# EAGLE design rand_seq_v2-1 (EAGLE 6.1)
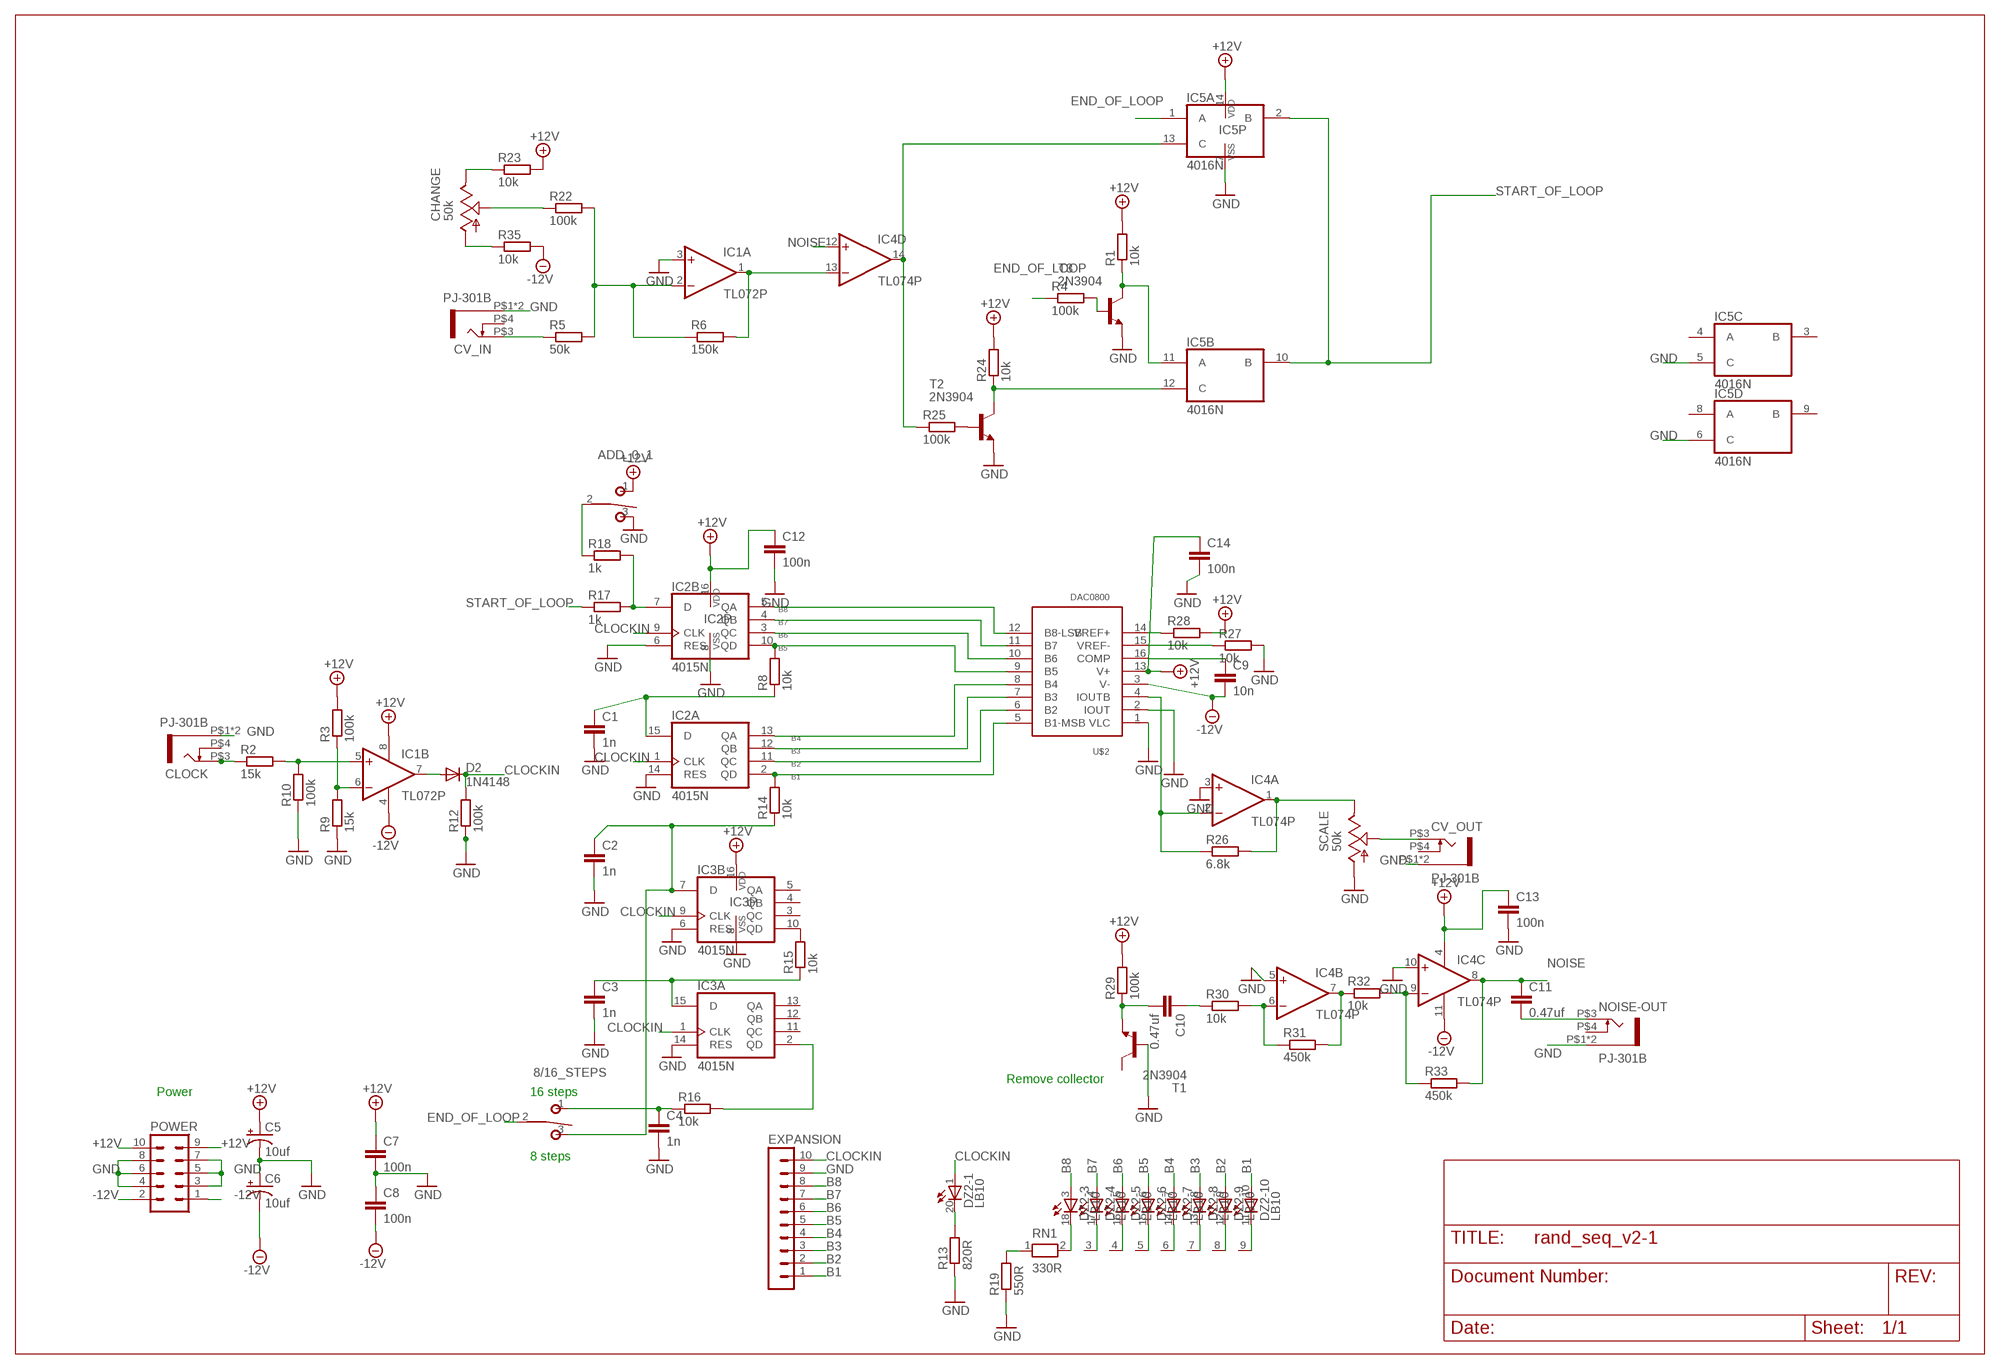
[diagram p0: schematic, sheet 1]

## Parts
8/16_STEPS  T-80-T-SPDT  [M9040P]
ADD_0_1  T-80-T-SPDT-ON-OFF-ON  [M9040P]
C1  1n  C-EU025-024X044  [C025-024X044]
C2  1n  C-EU025-024X044  [C025-024X044]
C3  1n  C-EU025-024X044  [C025-024X044]
C4  1n  C-EU025-024X044  [C025-024X044]
C5  10uf  CAP_POLPTH2  [CPOL-RADIAL-10UF-25V]
C6  10uf  CAP_POLPTH2  [CPOL-RADIAL-10UF-25V]
C7  100n  C-EU050-024X044  [C050-024X044]
C8  100n  C-EU050-024X044  [C050-024X044]
C9  10n  C-EU025-024X044  [C025-024X044]
C10  0.47uf  C-EU050-035X075  [C050-035X075]
C11  0.47uf  C-EU050-035X075  [C050-035X075]
C12  100n  C-EU050-024X044  [C050-024X044]
C13  100n  C-EU050-024X044  [C050-024X044]
C14  100n  C-EU050-024X044  [C050-024X044]
CHANGE  50k  ALPHA-9MMF2A  [EVUF]
CLOCK  PJ-301B  [PJ-301B]
CV_IN  PJ-301B  [PJ-301B]
CV_OUT  PJ-301B  [PJ-301B]
D2  1N4148  1N4148DO35-7  [DO35-7]
DZ2  LB10  [LB10]
EXPANSION  MA10-1  [MA10-1]
IC1  TL072P  [DIL08]
IC2  4015N  [DIL16]
IC3  4015N  [DIL16]
IC4  TL074P  [DIL14]
IC5  4016N  [DIL14]
NOISE-OUT  PJ-301B  [PJ-301B]
POWER  10_PIN_HEADER  [MA05-2]
R1  10k  R-EU_0207/10  [0207/10]
R2  15k  R-EU_0207/10  [0207/10]
R3  100k  R-EU_0207/10  [0207/10]
R4  100k  R-EU_0207/10  [0207/10]
R5  50k  R-EU_0207/10  [0207/10]
R6  150k  R-EU_0207/10  [0207/10]
R8  10k  R-EU_0207/10  [0207/10]
R9  15k  R-EU_0207/10  [0207/10]
R10  100k  R-EU_0207/10  [0207/10]
R12  100k  R-EU_0207/10  [0207/10]
R13  820R  R-EU_0207/10  [0207/10]
R14  10k  R-EU_0207/10  [0207/10]
R15  10k  R-EU_0207/10  [0207/10]
R16  10k  R-EU_0207/10  [0207/10]
R17  1k  R-EU_0207/10  [0207/10]
R18  1k  R-EU_0207/10  [0207/10]
R19  550R  R-EU_0207/2V  [0207/2V]
R22  100k  R-EU_0207/10  [0207/10]
R23  10k  R-EU_0207/10  [0207/10]
R24  10k  R-EU_0207/10  [0207/10]
R25  100k  R-EU_0207/10  [0207/10]
R26  6.8k  R-EU_0207/10  [0207/10]
R27  10k  R-EU_0207/10  [0207/10]
R28  10k  R-EU_0207/10  [0207/10]
R29  100k  R-EU_0207/10  [0207/10]
R30  10k  R-EU_0207/10  [0207/10]
R31  450k  R-EU_0207/10  [0207/10]
R32  10k  R-EU_0207/10  [0207/10]
R33  450k  R-EU_0207/10  [0207/10]
R35  10k  R-EU_0207/10  [0207/10]
RN1  330R  RN08  [RN-9]
SCALE  50k  ALPHA-9MMF2A  [EVUF]
T1  2N3904  [TO92]
T2  2N3904  [TO92]
T3  2N3904  [TO92]
U$2  DAC0800  [DIL16]

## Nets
+12V [power]: ADD_0_1.1(O) C5.1(+) C7.1 C12.1 C13.1 C14.1 IC1.8(P:V+) IC2.16(P:VDD) IC3.16(P:VDD) IC4.4(P:V+) IC5.14(P:VDD) POWER.9 POWER.10 R1.2 R3.2 R23.2 R24.2 R28.2 R29.2 U$2.13(V+)
-12V [power]: C6.2(-) C8.2 C9.2 IC1.4(P:V-) IC4.11(P:V-) POWER.1 POWER.2 R35.2 U$2.3(V-)
B1: DZ2.10(-10:A) EXPANSION.1 IC2.2(A:QD) R14.2 U$2.5(B1-MSB)
B2: DZ2.9(-9:A) EXPANSION.2 IC2.11(A:QC) U$2.6(B2)
B3: DZ2.8(-8:A) EXPANSION.3 IC2.12(A:QB) U$2.7(B3)
B4: DZ2.7(-7:A) EXPANSION.4 IC2.13(A:QA) U$2.8(B4)
B5: DZ2.6(-6:A) EXPANSION.5 IC2.10(B:QD) R8.2 U$2.9(B5)
B6: DZ2.5(-5:A) EXPANSION.6 IC2.3(B:QC) U$2.10(B6)
B7: DZ2.4(-4:A) EXPANSION.7 IC2.4(B:QB) U$2.11(B7)
B8: DZ2.3(-3:A) EXPANSION.8 IC2.5(B:QA) U$2.12(B8-LSB)
CLOCKIN: D2.C DZ2.1(-1:A) EXPANSION.10 IC2.1(A:CLK) IC2.9(B:CLK) IC3.1(A:CLK) IC3.9(B:CLK) R12.2
END_OF_LOOP: 8/16_STEPS.2(P) IC5.1(A:A) R4.1
GND [ground]: ADD_0_1.3(S) C1.2 C2.2 C3.2 C4.2 C5.2(-) C6.1(+) C7.2 C8.1 C12.2 C13.2 C14.2 CLOCK.P$1 CLOCK.P$2 CV_IN.P$1 CV_IN.P$2 CV_OUT.P$1 CV_OUT.P$2 EXPANSION.9 IC1.3(A:+IN) IC2.6(B:RES) IC2.8(P:VSS) IC2.14(A:RES) IC3.6(B:RES) IC3.8(P:VSS) IC3.14(A:RES) IC4.3(A:+IN) IC4.5(B:+IN) IC4.10(C:+IN) IC5.5(C:C) IC5.6(D:C) IC5.7(P:VSS) NOISE-OUT.P$1 NOISE-OUT.P$2 POWER.3 POWER.4 POWER.5 POWER.6 POWER.7 POWER.8 R9.1 R10.1 R12.1 R13.1 R19.1 R27.2 SCALE.1(A) T1.2(B) T2.3(E) T3.3(E) U$2.1(VLC) U$2.2(IOUT)
MAIN_OUT: IC4.1(A:OUT) R26.2 SCALE.3(E)
N$1: R4.2 T3.2(B)
N$2: CLOCK.P$3 R2.1
N$3: CV_IN.P$3 R5.1
N$4: IC5.11(B:A) R1.1 T3.1(C)
N$5: IC1.5(B:+IN) R2.2 R10.2
N$6: IC1.2(A:-IN) R5.2 R6.1 R22.2
N$7: IC1.1(A:OUT) IC4.13(D:-IN) R6.2
N$8: D2.A IC1.7(B:OUT)
N$9: 8/16_STEPS.3(S) C2.1 IC3.7(B:D) R14.1
N$10: C1.1 IC2.15(A:D) R8.1
N$11: ADD_0_1.2(P) R18.1
N$12: IC1.6(B:-IN) R3.1 R9.2
N$13: IC4.2(A:-IN) R26.1 U$2.4(IOUTB)
N$14: IC3.10(B:QD) R15.2
N$15: C11.2 NOISE-OUT.P$3
N$16: C10.2 R29.1 T1.3(E)
N$17: 8/16_STEPS.1(O) C4.1 R16.1
N$18: C3.1 IC3.15(A:D) R15.1
N$19: IC2.7(B:D) R17.2 R18.2
N$20: C10.1 R30.1
N$21: IC4.6(B:-IN) R30.2 R31.1
N$22: IC4.7(B:OUT) R31.2 R32.1
N$23: R27.1 U$2.15(VREF-)
N$24: IC4.14(D:OUT) IC5.13(A:C) R25.1
N$25: C9.1 U$2.16(COMP)
N$26: R28.1 U$2.14(VREF+)
N$27: IC4.9(C:-IN) R32.2 R33.1
N$28: DZ2.20(-1:C) R13.2
N$29: IC3.2(A:QD) R16.2
N$30: DZ2.18(-3:C) RN1.2
N$31: DZ2.17(-4:C) RN1.3
N$32: DZ2.16(-5:C) RN1.4
N$33: DZ2.15(-6:C) RN1.5
N$34: DZ2.14(-7:C) RN1.6
N$35: DZ2.13(-8:C) RN1.7
N$36: DZ2.12(-9:C) RN1.8
N$37: DZ2.11(-10:C) RN1.9
N$38: R19.2 RN1.1
N$39: CV_OUT.P$3 SCALE.2(S)
N$43: CHANGE.2(S) R22.1
N$44: R25.2 T2.2(B)
N$45: IC5.12(B:C) R24.1 T2.1(C)
N$47: CHANGE.3(E) R23.1
N$48: CHANGE.1(A) R35.1
NOISE: C11.1 IC4.8(C:OUT) IC4.12(D:+IN) R33.2
START_OF_LOOP: IC5.2(A:B) IC5.10(B:B) R17.1
Unconnected: CLOCK.P$4 CV_IN.P$4 CV_OUT.P$4 DZ2.2(-2:A) DZ2.19(-2:C) IC3.3(B:QC) IC3.4(B:QB) IC3.5(B:QA) IC3.11(A:QC) IC3.12(A:QB) IC3.13(A:QA) IC5.3(C:B) IC5.4(C:A) IC5.8(D:A) IC5.9(D:B) NOISE-OUT.P$4 T1.1(C)

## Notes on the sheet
- /Users/aash/Dropbox/Electronics/!MODULAR/design/logo copy.bmp
- Remove collector
- Power | 16 steps
- 8 steps

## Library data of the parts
8/16_STEPS = TomW:T-80-T-SPDT
ADD_0_1 = TomW:T-80-T-SPDT-ON-OFF-ON
C1-C4 C7-C9 C12-C14 = TomW:C-EU: CAPACITOR, European symbol
C5 C6 = SparkFun-Passives:CAP_POL: Capacitor Polarized
C10 C11 = rcl:C-EU: CAPACITOR, European symbol
CHANGE SCALE = TomW:ALPHA-9MM: 9 mm Square Rotary Potentiometers Source: Panasonic
CLOCK CV_IN CV_OUT NOISE-OUT = TomW:PJ-301B
D2 = diode:1N4148: DIODE
DZ2 = led:LB10: LED BLOCK 10-LED bar graph, DIL, Siemens
EXPANSION = con-lstb:MA10-1: PIN HEADER; OC_FARNELL: unknown; OC_NEWARK: unknown
IC1 = TomW:TL072: OP AMP
IC2 IC3 = 40xx:4015: Dual 4-bit static SHIFT REGISTER
IC4 = linear:TL074: OP AMP
IC5 = 40xx:4016: Quad bilateral ANALOG SWITCH
POWER = TomW:10_PIN_HEADER: PIN HEADER; OC_FARNELL: unknown; OC_NEWARK: unknown
R1-R6 R8-R10 R12-R18 R22-R33 R35 = TomW:R-EU_: RESISTOR, European symbol
R19 = rcl:R-EU_: RESISTOR, European symbol
RN1 = TomW:RN08: RESISTOR NETWORK; OC_FARNELL: unknown; OC_NEWARK: unknown
T1-T3 = transistor:2N3904: NPN TRANSISTOR
U$2 = TomW:DAC0800

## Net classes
0 default: width 0.254 mm
1 power: width 0.61 mm
2 ground: width 0.61 mm

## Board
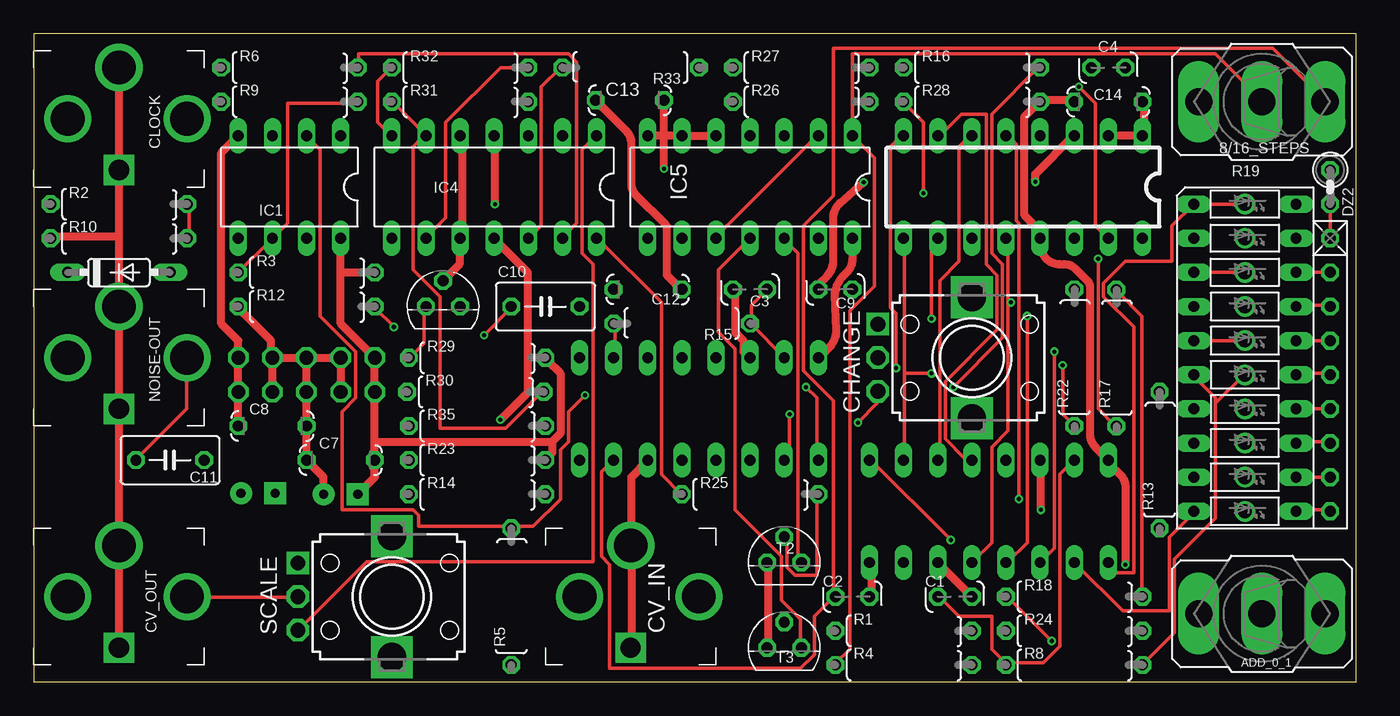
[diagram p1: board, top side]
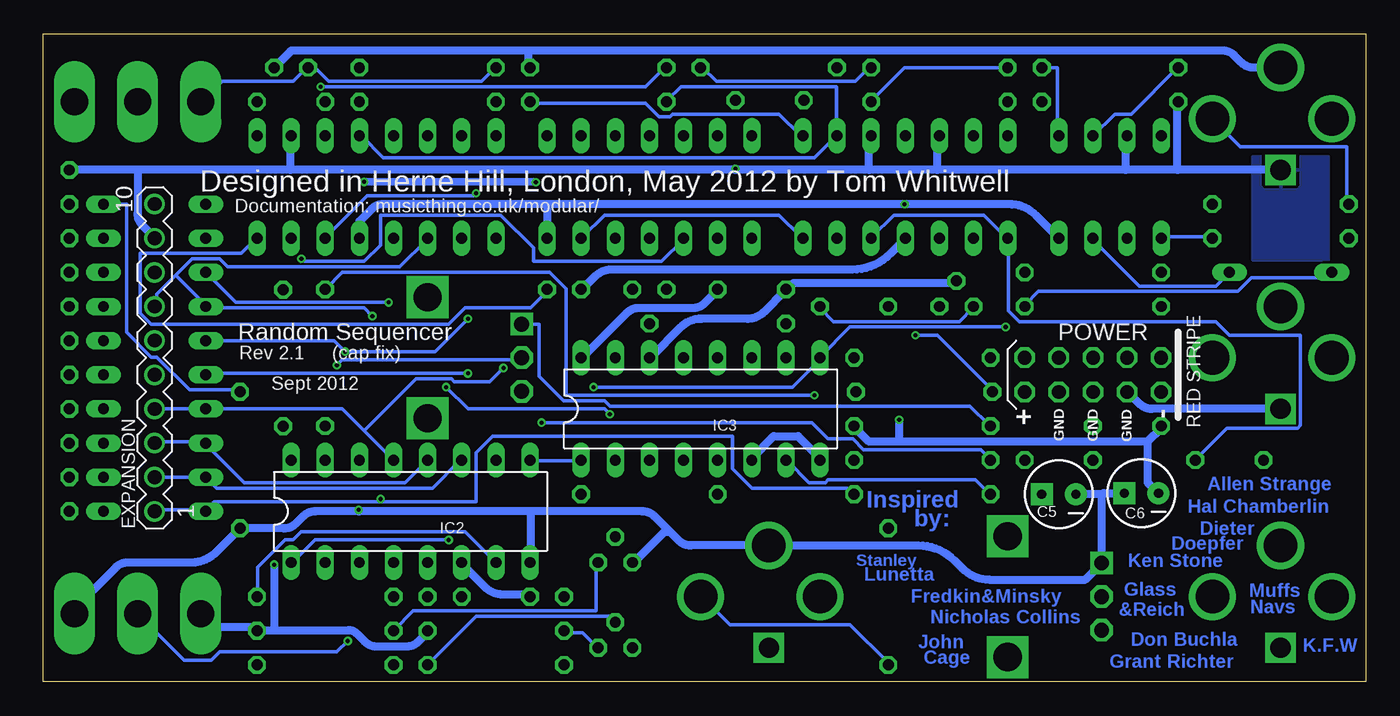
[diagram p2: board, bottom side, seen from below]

Size 98.48 x 48.25 mm. Coordinates in mm from the lower left corner, seen from the top.
Outline: 0,0 98.48,0 98.48,48.25 0,48.25 0,0
Copper layers (1*16): Top 0.035mm / dielectric 1.5mm / Bottom 0.035mm
Design rules: minimum track width 6mil, minimum drill 12mil, track to track 6mil, track to pad 6mil, pad to pad 6mil, via to via 6mil, smd to smd 0mil, copper to edge 10mil, drill to drill 10mil, minimum pad ring 10mil, minimum via ring 6mil, stop-mask expansion 2mil, vias tented up to drill 100mil, thermal gap 10mil

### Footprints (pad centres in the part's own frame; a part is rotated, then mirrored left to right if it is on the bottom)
M9040P = drill 2.03 long: 1 0,4.699; 2 0,0; 3 0,-4.699
C025-024X044 = drill 0.813 octagon: 1 -1.27,0; 2 1.27,0
CPOL-RADIAL-10UF-25V = drill 0.7 pad 1.651 square: 1 1.27,0 | drill 0.7 pad 1.651: 2 -1.27,0
C050-024X044 = drill 0.813 octagon: 1 -2.54,0; 2 2.54,0
C050-035X075 = drill 0.813 octagon: 1 -2.54,0; 2 2.54,0
EVUF = drill 1.1 pad 1.676 square: 1 -2.5,-7 | drill 1.1 pad 1.676 octagon: 2 0,-7; 3 2.5,-7 | drill 2.1 pad 2.8 square: M1 4.5,0; M2 -4.5,0
PJ-301B = drill 1.5 square: P$1 3.81,0 | drill 2.5: P$2 -3.81,0; P$3 0,5.08; P$4 0,-3.81
DO35-7 = drill 0.813 long: A 3.81,0; C -3.81,0
LB10 = drill 0.813 long: 1 -11.43,-3.81; 2 -8.89,-3.81; 3 -6.35,-3.81; 4 -3.81,-3.81; 5 -1.27,-3.81; 6 1.27,-3.81; 7 3.81,-3.81; 8 6.35,-3.81; 9 8.89,-3.81; 10 11.43,-3.81; 11 11.43,3.81; 12 8.89,3.81; 13 6.35,3.81; 14 3.81,3.81; 15 1.27,3.81; 16 -1.27,3.81; 17 -3.81,3.81; 18 -6.35,3.81; 19 -8.89,3.81; 20 -11.43,3.81
MA10-1 = drill 1.016: 1 -11.43,0; 2 -8.89,0; 3 -6.35,0; 4 -3.81,0; 5 -1.27,0; 6 1.27,0; 7 3.81,0; 8 6.35,0; 9 8.89,0; 10 11.43,0
DIL08 = drill 0.813 pad 1.27 long: 1 -3.81,-3.81; 2 -1.27,-3.81; 3 1.27,-3.81; 4 3.81,-3.81; 5 3.81,3.81; 6 1.27,3.81; 7 -1.27,3.81; 8 -3.81,3.81
DIL16 = drill 0.813 long: 1 -8.89,-3.81; 2 -6.35,-3.81; 3 -3.81,-3.81; 4 -1.27,-3.81; 5 1.27,-3.81; 6 3.81,-3.81; 7 6.35,-3.81; 8 8.89,-3.81; 9 8.89,3.81; 10 6.35,3.81; 11 3.81,3.81; 12 1.27,3.81; 13 -1.27,3.81; 14 -3.81,3.81; 15 -6.35,3.81; 16 -8.89,3.81
DIL14 = drill 0.813 long: 1 -7.62,-3.81; 2 -5.08,-3.81; 3 -2.54,-3.81; 4 0,-3.81; 5 2.54,-3.81; 6 5.08,-3.81; 7 7.62,-3.81; 8 7.62,3.81; 9 5.08,3.81; 10 2.54,3.81; 11 0,3.81; 12 -2.54,3.81; 13 -5.08,3.81; 14 -7.62,3.81
MA05-2 = drill 1.016 octagon: 1 -5.08,-1.27; 2 -5.08,1.27; 3 -2.54,-1.27; 4 -2.54,1.27; 5 0,-1.27; 6 0,1.27; 7 2.54,-1.27; 8 2.54,1.27; 9 5.08,-1.27; 10 5.08,1.27
0207/10 = drill 0.813 octagon: 1 -5.08,0; 2 5.08,0
0207/2V = drill 0.813 octagon: 1 -1.27,0; 2 1.27,0
RN-9 = drill 0.813 octagon: 1 -10.16,0; 2 -7.62,0; 3 -5.08,0; 4 -2.54,0; 5 0,0; 6 2.54,0; 7 5.08,0; 8 7.62,0; 9 10.16,0
TO92 = drill 0.813 octagon: 1 1.27,0; 2 0,1.905; 3 -1.27,0

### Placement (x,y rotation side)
8/16_STEPS  91.44,43.18 90 top
ADD_0_1  91.44,5.08 90 top
C1  68.58,6.35 0 top
C2  60.96,6.35 0 top
C3  53.34,29.21 180 top
C4  80.01,45.72 0 top
C5  22.86,13.97 180 bottom
C6  16.71,14.05 180 bottom
C7  22.86,16.51 180 top
C8  17.78,19.05 180 top
C9  59.69,29.21 180 top
C10  38.1,27.94 0 top
C11  10.16,16.51 180 top
C12  45.72,29.21 180 top
C13  44.39,43.29 0 top
C14  80.01,43.18 0 top
CHANGE  69.85,24.13 270 top
CLOCK  6.35,41.91 270 top
CV_IN  44.45,6.35 270 top
CV_OUT  6.35,6.35 270 top
D2  6.35,30.48 0 top
DZ2  90.17,24.13 270 top
EXPANSION  90.17,24.13 90 bottom
IC1  19.05,36.83 180 top
IC2  71.12,12.7 0 bottom
IC3  49.53,20.32 0 bottom
IC4  34.29,36.83 180 top
IC5  53.34,36.83 180 top
NOISE-OUT  6.35,24.13 270 top
POWER  20.32,22.86 180 bottom
R1  64.77,3.81 0 top
R2  6.35,35.56 0 top
R3  20.32,30.48 0 top
R4  64.77,1.27 0 top
R5  35.56,6.35 90 top
R6  19.05,45.72 0 top
R8  77.47,1.27 0 top
R9  19.05,43.18 0 top
R10  6.35,33.02 0 top
R12  20.32,27.94 0 top
R13  83.82,16.51 90 top
R14  33.02,13.97 0 top
R15  48.26,26.67 180 top
R16  69.85,45.72 0 top
R17  80.61,24.1 90 top
R18  77.47,6.35 0 top
R19  96.52,36.83 270 top
R22  77.48,24.13 90 top
R23  33.02,16.51 0 top
R24  77.47,3.81 0 top
R25  53.34,13.97 0 top
R26  57.15,43.18 0 top
R27  57.15,45.72 0 top
R28  69.85,43.18 0 top
R29  33.02,24.13 0 top
R30  32.89,21.59 0 top
R31  31.75,43.18 0 top
R32  31.75,45.72 0 top
R33  44.45,45.72 180 top
R35  33.02,19.05 0 top
RN1  96.52,22.86 270 top
SCALE  26.67,6.35 270 top
T1  30.48,27.94 0 top
T2  55.88,8.89 0 top
T3  55.88,2.54 0 top
U$2  73.66,36.83 180 top

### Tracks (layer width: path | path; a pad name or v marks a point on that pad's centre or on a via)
+12V  (via drill 0.3)
  Top 0.61: C5.1 25.4,15.24 C7.1 25.4,17.88 | 25.4,17.88 POWER.10 POWER.9 22.86,26.67 22.86,30.48 | 22.86,30.48 IC1.8 | IC5.14 60.96,31.52 arc-45 60.51,30.44 60.36,30.29 arc45 59.63,28.76 59.74,26.16 arc-45 59.2,24.86 58.52,24.18 IC3.16 | C13.1 44.11,41.03 arc-45 44.5,40.09 44.5,37.09 arc45 44.87,36.21 47.03,34.05 arc-45 47.14,33.77 47.14,30.28 48.16,29.26 C12.1 | 38.61,17.88 38.61,17.07 38.2,16.66 R23.2 | 38.61,17.88 39.22,18.49 39.22,22.96 38.2,23.98 R29.2 | C14.1 77.42,43.28 74.98,43.28 R28.2 74.78,43.08 73.76,42.06 73.76,34.75 74.78,33.73 74.78,33.12 U$2.13 74.98,32.92 74.98,32.48 arc90 76.37,31.09 76.72,31.09 arc-45 77.56,30.74 78.5,29.8 arc-45 78.64,29.47 78.64,18.45 arc45 79.04,17.48 IC2.16 80.06,16.26 80.9,15.41 arc-45 81.28,14.5 v81.28,8.74 | 22.86,30.48 R3.2 | v34.34,35.56 34.34,40.64 IC4.4 | 25.4,17.88 38.61,17.88
  Bottom 0.61: IC1.8 24.57,34.73 arc-45 26.58,35.56 v34.34,35.56 60.96,35.56 | 60.96,35.56 73.13,35.56 arc-45 74.03,35.19 74.93,34.29 U$2.13 | C12.1 48.36,29.06 49.22,28.2 arc45 50.09,27.84 54.11,27.84 arc-45 55.05,27.45 58.32,24.18 IC3.16 | 81.28,3.86 75.72,3.86 arc45 75.15,3.62 74.54,3.02 arc-45 73.64,2.64 71.41,2.64 arc-45 70.57,2.99 69.9,3.66 R1.2 | 81.28,3.86 82.5,3.86 R24.2 82.7,4.06 85.55,4.06 86.56,5.08 ADD_0_1.1 | v81.28,8.74 81.28,3.86 | 60.96,35.56 IC5.14
-12V  (via drill 0.3)
  Top 0.61: C8.2 POWER.2 POWER.1 15.24,25.4 13.97,26.67 13.97,39.37 IC1.4 | v74.58,37.21 74.57,37.8 77.42,40.64 U$2.3 | v61.8,37.2 60.02,35.64 arc45 59.54,34.46 59.54,31.32 arc-45 59.09,30.23 58.52,29.67 58.52,29.26 C9.2 | v34.75,19.51 36.78,21.54 36.78,30.48 34.34,32.92 IC4.11
  Bottom 0.61: 16.26,17.88 34.75,17.88 | 34.75,17.88 36.98,17.88 38,18.9 R35.2 | 16.26,17.88 15.24,18.9 C8.2 | C9.2 58.32,29.26 57.42,30.16 arc45 56.16,30.68 38.26,30.68 arc-45 35.38,31.88 34.34,32.92 IC4.11 | v61.8,37.2 v74.58,37.21 | v34.75,19.51 34.75,17.88 | 16.26,17.88 16.26,14.86 C6.2
B1  (via drill 0.3)
  Top 0.254: v73.36,13.61 73.36,34.14 73.15,34.34 73.15,40.03 72.54,40.64 U$2.5 | IC2.2 77.62,8.74 81.08,5.28 84.53,5.28 84.53,10.77 86.36,12.6 DZ2.10
  Bottom 0.254: 73.36,13.41 85.75,13.41 86.36,12.8 | 73.36,13.41 66.24,13.41 66.24,17.07 65.02,18.29 47.14,18.29 47.14,15.85 45.72,14.43 38.61,14.43 38.2,14.02 R14.2 | 86.36,12.8 DZ2.10 86.36,12.8 | 73.36,13.41 v73.36,13.61 | 86.36,12.8 90.02,12.8 EXPANSION.1
B2
  Top 0.254: U$2.6 69.7,40.64 68.89,39.83 68.89,31.29 67.46,29.87 67.46,16.66 IC2.11
  Bottom 0.254: IC2.11 67.46,16.46 69.49,14.43 85.55,14.43 DZ2.9 90.02,15.24 EXPANSION.2
B3
  Top 0.254: U$2.7 67.46,40.64 69.09,42.27 70.92,42.27 70.92,31.09 71.73,30.28 71.73,26.21 67.87,22.35 67.87,18.09 69.29,16.66 69.7,16.66 IC2.12
  Bottom 0.254: IC2.12 69.9,16.46 71.53,14.83 83.52,14.83 86.36,17.68 DZ2.8 86.36,17.88 90.02,17.88 EXPANSION.3
B4  (via drill 0.3)
  Top 0.254: v64.21,23.37 64.21,27.43 63.8,27.84 63.8,39.83 64.62,40.64 U$2.8
  Bottom 0.254: 74.57,18.69 76.2,20.32 DZ2.7 90.02,20.32 EXPANSION.4 | 74.57,18.69 72.54,16.66 IC2.13 | v64.21,23.37 65.23,22.35 67.87,22.35 68.07,22.55 70.71,22.55 74.57,18.69
B5  (via drill 0.3)
  Top 0.254: 64.82,22.96 64.82,32.92 U$2.9 | 64.82,22.96 64.82,16.66 IC2.10 | 87.99,20.73 87.99,21.13 86.36,22.76 DZ2.6 | 87.99,20.73 87.99,12.19 84.94,9.14 84.94,3.66 82.7,1.42 R8.2 | 87.99,20.73 90.02,22.76 EXPANSION.5 | v66.85,22.96 64.82,22.96
  Bottom 0.254: v66.85,22.96 86.36,22.96 DZ2.6
B6  (via drill 0.3)
  Top 0.254: v76,24.59 76,9.96 74.98,8.94 IC2.3 | v66.85,27.03 66.85,32.51 67.26,32.92 U$2.10 | DZ2.5 90.02,25.4 EXPANSION.6
  Bottom 0.254: DZ2.5 76.81,25.4 v76,24.59 69.29,24.59 v66.85,27.03
B7  (via drill 0.3)
  Top 0.254: v73.97,27.23 73.97,10.36 72.54,8.94 IC2.4
  Bottom 0.254: 88.59,30.28 90.02,28.85 90.02,28.04 EXPANSION.7 | 88.59,30.28 87.38,31.5 85.34,31.5 84.73,30.89 71.93,30.89 69.9,32.92 U$2.11 | v73.97,27.23 74.57,27.84 86.36,27.84 DZ2.4 86.36,28.04 88.59,30.28
B8  (via drill 0.3)
  Top 0.254: DZ2.3 90.02,30.48 EXPANSION.8 | 72.54,28.25 72.54,32.92 U$2.12 | 72.54,28.25 72.54,18.69 71.32,17.48 71.32,10.36 69.9,8.94 IC2.5 | 72.54,28.25 v72.75,28.25
  Bottom 0.254: DZ2.3 84.12,28.25 v72.75,28.25
CLOCKIN  (via drill 0.3)
  Top 0.254: v26.82,26.42 25.4,27.84 R12.2 | IC2.1 80.06,8.74 80.67,8.13 81.89,8.13 81.89,26.42 79.65,28.65 79.65,29.67 81.28,31.29 84.73,31.29 84.73,33.93 DZ2.1 90.02,35.56 EXPANSION.10 | v68.28,10.57 62.38,16.46 IC2.9 | v57.51,21.95 58.32,21.13 58.32,16.66 IC3.1
  Bottom 0.254: D2.C 2.64,30.48 3.05,30.07 8.53,30.07 9.55,29.06 24.38,29.06 25.4,28.04 R12.2 | v26.82,26.42 38.41,26.42 40.64,24.18 IC3.9 40.64,23.98 42.67,21.95 v57.51,21.95 | IC3.1 58.52,16.46 62.18,16.46 IC2.9 | v68.28,10.57 78.23,10.57 79.86,8.94 IC2.1
END_OF_LOOP
  Top 0.254: R4.1 59.74,1.42 60.76,2.44 60.76,27.64 62.59,29.46 62.59,39.01 IC5.1 60.96,46.74 87.99,46.74 91.44,43.28 8/16_STEPS.2
GND  (via drill 0.3)
  Top 0.61: CLOCK.P$2 6.35,38.2 | 6.35,38.2 CLOCK.P$1 | CLOCK.P$1 6.35,33.12 | 6.35,33.12 6.35,28.04 | 6.35,28.04 NOISE-OUT.P$2 | NOISE-OUT.P$2 NOISE-OUT.P$1 | NOISE-OUT.P$1 CV_OUT.P$2 CV_OUT.P$1 | C5.2 21.59,15.24 C7.2 C8.1 POWER.6 POWER.5 | POWER.4 POWER.3 | POWER.3 POWER.5 | POWER.5 POWER.7 POWER.8 | IC3.14 53.24,24.18 52.83,24.59 52.83,25.4 52.22,26.01 52.22,29.06 C3.2 | T1.2 30.48,29.87 31.7,31.09 31.7,32.92 IC4.10 31.9,33.12 31.9,40.64 IC4.5 | 46.94,40.64 IC5.6 IC5.5 | 46.94,40.64 IC5.7 | 46.94,40.64 C13.2 | U$2.2 U$2.1 82.7,40.84 82.7,43.08 C14.2 | v46.94,38.2 46.94,40.64 | T3.3 54.66,2.64 54.66,8.74 T2.3 | IC2.6 C1.2 | C2.2 62.38,6.5 62.38,8.74 IC2.8 | R12.1 15.24,27.84 17.68,25.4 17.68,24.18 POWER.3 | 20.32,24.18 POWER.5 | v74.98,12.8 74.98,16.46 IC2.14 | IC3.6 45.72,16.46 44.5,15.24 44.5,10.16 CV_IN.P$2 44.5,9.96 44.5,2.64 CV_IN.P$1 | 6.35,33.12 1.42,33.12 R10.1 | 6.3,20.32 NOISE-OUT.P$1 | NOISE-OUT.P$2 6.3,28.04 6.35,28.04 | CLOCK.P$1 6.3,38.2 6.35,38.2
  Bottom 0.61: CLOCK.P$1 14.02,38.1 | 14.02,38.1 17.88,38.1 | 17.88,38.1 31.9,38.1 | 31.9,38.1 36.98,38.1 | 36.98,38.1 46.94,38.1 | 46.94,38.1 80.06,38.1 | 80.06,38.1 91.44,38.1 | 91.44,38.1 R19.1 | 51.92,11.28 51.17,10.53 arc-45 50.27,10.16 CV_IN.P$2 33.33,10.16 arc45 30.63,9.04 30.04,8.45 arc-45 28.03,7.62 20.9,7.62 SCALE.1 19.66,13.91 | 51.92,11.28 52.97,12.33 arc-45 53.87,12.7 62.18,12.7 | 62.18,12.7 74.98,12.7 | 74.98,12.7 78.21,12.7 arc-45 79.11,12.33 79.64,11.8 arc45 80.54,11.43 R13.1 85.62,9.63 arc45 87.41,8.89 92.18,8.89 arc-45 93.08,8.52 96.52,5.08 ADD_0_1.3 | CLOCK.P$2 8.36,45.72 arc45 9.26,46.09 9.79,46.62 arc-45 10.69,46.99 62.38,46.99 | 62.38,46.99 80.01,46.99 80.01,46.94 arc-45 80.1,46.9 C4.2 | T1.2 30.48,29.67 42.67,29.67 43.08,29.26 C12.2 43.28,29.06 44.81,27.53 arc45 46.02,27.03 49.5,27.03 arc-45 51.03,26.39 53.24,24.18 IC3.14 | 17.88,38.1 17.88,40.64 IC1.3 | 31.9,38.1 31.9,40.64 IC4.5 | 36.98,38.1 36.98,40.64 IC4.3 | 14.02,38.1 14.02,43.08 R9.1 | 91.44,38.1 91.44,34.87 arc-45 91.07,33.97 90.22,33.12 EXPANSION.9 | 80.06,38.1 80.06,40.64 U$2.2 | v46.94,38.2 46.94,38.1 | IC3.8 40.64,16.66 42.27,18.29 44.09,18.29 45.72,16.66 IC3.6 | v74.98,12.8 74.98,12.7 | 62.18,12.7 62.18,8.94 IC2.8 | IC2.6 67.26,8.74 65.58,7.06 arc-45 64.24,6.5 62.38,6.5 C2.2 | T2.3 54.46,8.94 52.22,11.18 52.02,11.18 51.92,11.28 | 62.38,46.99 62.38,45.72 R27.2 | NOISE-OUT.P$1 15.95,20.32 arc45 16.82,20.68 17.68,21.54 POWER.4 | 19.66,13.91 19.53,14.05 C6.1 | 19.66,13.91 19.71,13.97 C5.2
  pour Bottom: 2.79,39.07 8.41,39.09 8.41,31.42 2.79,31.42
MAIN_OUT
  Top 0.254: SCALE.3 19.71,3.86 24.79,8.94 41.66,8.94 41.66,31.09 40.84,31.9 40.84,39.62 41.86,40.64 IC4.1
  Bottom 0.254: IC4.1 42.06,40.64 43.69,42.27 51.61,42.27 51.82,42.06 52.63,42.06 53.65,43.08 62.18,43.08 R26.2
N$1
  Bottom 0.254: T3.2 55.88,4.47 56.29,4.88 66.24,4.88 69.7,1.42 R4.2
N$2
  Top 0.254: 11.38,42.06 CLOCK.P$3 11.38,42.06
  Bottom 0.254: R2.1 1.42,35.56 1.42,39.83 9.35,39.83 11.38,41.86 CLOCK.P$3
N$3
  Bottom 0.254: R5.1 35.56,1.42 38.41,4.27 47.35,4.27 49.38,6.3 CV_IN.P$3
N$4
  Top 0.254: IC5.11 53.24,32.92 51,30.68 51,26.01 52.22,24.79 52.22,12.8 55.68,9.35 55.68,6.1 57.1,4.67 57.1,2.64 T3.1
  Bottom 0.254: T3.1 57.3,2.64 58.32,3.66 59.54,3.66 R1.1
N$5
  Top 0.254: R10.2 11.58,33.12 11.58,35.56 R2.2
  Bottom 0.254: IC1.5 15.24,33.12 11.58,33.12 R10.2
N$6  (via drill 0.3)
  Top 0.254: 35.56,11.58 28.65,11.58 28.65,12.39 28.25,12.8 22.96,12.8 22.96,20.12 23.98,21.13 23.98,24.59 21.34,27.23 21.34,39.62 IC1.2 | 35.56,11.58 R5.2 35.56,11.58 | v41.05,21.34 39.83,20.12 39.83,17.88 39.22,17.27 39.22,13.61 37.19,11.58 35.56,11.58
  Bottom 0.254: IC1.2 18.69,42.27 17.48,42.27 14.02,45.72 R6.1 | v41.05,21.34 59.54,21.34 59.54,29.26 60.76,30.48 76.2,30.48 77.42,29.26 R22.2
N$7
  Top 0.254: IC4.13 39.42,33.12 40.44,34.14 40.44,46.13 39.83,46.74 24.18,46.74 24.18,45.72 R6.2
  Bottom 0.254: IC1.1 22.96,40.64 22.96,45.72 23.98,45.72 R6.2
N$8
  Bottom 0.254: D2.A 11.18,29.46 16.87,29.46 20.32,32.92 IC1.7
N$9
  Top 0.254: IC3.7 43.08,16.46 42.27,15.65 42.27,9.35 42.88,8.74 42.88,1.02 57.1,1.02 58.12,2.03 58.12,4.88 59.54,6.3 C2.1 59.54,6.5 59.54,20.93 57.3,23.16 57.3,33.93 59.54,36.17 59.54,47.14 92.25,47.14 96.11,43.28 8/16_STEPS.3
  Bottom 0.254: R14.1 28.04,14.02 29.06,15.04 40.03,15.04 40.23,14.83 41.45,14.83 43.08,16.46 IC3.7
N$10
  Top 0.254: C1.1 67.46,6.3 68.89,4.88 71.32,4.88 71.32,2.44 72.34,1.42 R8.1 72.54,1.42 75.18,1.42 76.4,2.64 76.4,15.44 77.42,16.46 IC2.15
N$11  (via drill 0.3)
  Top 0.254: v75.79,3.05 72.54,6.3 R18.1
  Bottom 0.254: v75.79,3.05 76.61,2.23 85.34,2.23 85.95,1.63 87.99,1.63 ADD_0_1.2
N$12
  Top 0.254: R3.1 17.68,32.92 IC1.6 17.88,33.12 18.9,34.14 18.9,43.08 23.98,43.08 R9.2
N$13
  Bottom 0.254: 39.42,40.64 39.42,44.3 51,44.3 52.02,43.28 R26.1 | 39.42,40.64 IC4.2 39.42,40.64 | 39.42,40.64 41.05,39.01 73.15,39.01 74.78,40.64 U$2.4
N$14
  Top 0.254: IC3.10 43.28,24.18 43.28,26.62 R15.2
N$15
  Top 0.254: C11.2 7.72,16.66 11.38,20.32 11.38,23.98 NOISE-OUT.P$3
N$16
  Top 0.254: R29.1 28.04,24.18 29.06,25.2 29.06,27.84 T1.3
  Bottom 0.254: C10.2 40.64,27.84 39.62,26.82 30.28,26.82 29.26,27.84 T1.3
N$17
  Bottom 0.254: R16.1 64.82,45.72 65.84,44.7 77.22,44.7 78.23,45.72 78.64,45.72 C4.1 78.84,45.72 79.86,44.7 85.14,44.7 86.56,43.28 8/16_STEPS.1
N$18
  Top 0.254: IC3.15 55.88,24.18 53.44,26.62 R15.1 53.44,26.82 53.44,28.04 54.46,29.06 C3.1
N$19
  Top 0.254: R17.2 80.67,29.06 82.5,27.23 82.5,6.5 R18.2
  Bottom 0.254: IC2.7 64.82,8.94 67.06,11.18 79.25,11.18 79.86,10.57 80.47,10.57 82.5,8.53 82.5,6.5 R18.2
N$20  (via drill 0.3)
  Top 0.254: v33.53,25.81 35.56,27.84 C10.1
  Bottom 0.254: v33.53,25.81 31.9,25.81 27.84,21.74 R30.1
N$21
  Top 0.254: 29.06,40.64 28.25,39.83 28.25,30.68 30.28,28.65 30.28,18.9 35.15,18.9 37.8,21.54 R30.2 | 29.06,40.64 IC4.6 29.06,40.64 | 29.06,40.64 29.06,40.84 26.82,43.08 R31.1
N$22
  Top 0.254: IC4.7 26.62,40.64 25.6,41.66 25.6,44.7 26.62,45.72 R32.1
  Bottom 0.254: R31.2 36.78,43.28 34.34,45.72 26.82,45.72 R32.1
N$23  (via drill 0.3)
  Top 0.254: v77.83,44.3 79.05,43.08 79.05,33.93 79.86,33.12 U$2.15
  Bottom 0.254: v77.83,44.3 53.65,44.3 52.22,45.72 R27.1
N$24
  Top 0.254: R25.1 48.16,14.02 46.74,15.44 46.74,28.25 42.06,32.92 IC4.14
  Bottom 0.254: IC5.13 58.32,33.12 56.69,34.75 43.69,34.75 42.06,33.12 IC4.14
N$25
  Bottom 0.254: C9.1 60.96,29.06 62.18,27.84 67.06,27.84 68.28,26.62 90.42,26.62 91.24,27.43 91.24,31.9 83.72,31.9 82.7,32.92 U$2.16
N$26  (via drill 0.3)
  Top 0.254: v66.24,36.37 66.24,41.66 64.82,43.08 R28.1
  Bottom 0.254: v66.24,36.37 66.45,36.17 74.37,36.17 77.42,33.12 U$2.14
N$27
  Top 0.254: IC4.9 29.26,33.12 30.68,34.54 30.68,41.66 34.75,45.72 36.78,45.72 R32.2
  Bottom 0.254: R33.1 49.38,45.72 48.36,44.7 38,44.7 36.98,45.72 R32.2
N$28
  Bottom 0.254: R13.2 83.92,21.74 87.58,21.74 90.02,24.18 90.42,24.18 92.25,26.01 92.25,35.56 93.88,35.56 DZ2.20
N$29  (via drill 0.3)
  Top 0.254: v56.29,19.91 56.29,17.07 55.88,16.66 IC3.2 | v68.48,21.95 72.14,25.6 72.14,31.09 71.32,31.9 71.32,42.27 74.78,45.72 R16.2
  Bottom 0.254: v56.29,19.91 56.69,20.32 66.85,20.32 v68.48,21.95
N$30
  Top 0.254: RN1.2 94.08,30.48 DZ2.18
N$31
  Top 0.254: DZ2.17 94.08,28.04 96.52,28.04 RN1.3
N$32
  Top 0.254: RN1.4 94.08,25.4 DZ2.16
N$33
  Top 0.254: DZ2.15 94.08,22.96 96.52,22.96 RN1.5
N$34
  Top 0.254: RN1.6 94.08,20.32 DZ2.14
N$35
  Top 0.254: DZ2.13 94.08,17.88 96.52,17.88 RN1.7
N$36
  Top 0.254: RN1.8 94.08,15.24 DZ2.12
N$37
  Top 0.254: DZ2.11 94.08,12.8 96.52,12.8 RN1.9
N$38
  Top 0.254: R19.2 96.52,33.12 RN1.1
N$39
  Top 0.254: SCALE.2 19.51,6.3 11.58,6.3 CV_OUT.P$3
N$43  (via drill 0.3)
  Top 0.254: v76.61,23.57 76.61,19.91 77.42,19.1 R22.1
  Bottom 0.254: v76.61,23.57 76.2,23.98 62.99,23.98 CHANGE.2
N$44
  Top 0.254: T2.2 55.88,10.77 56.08,10.57 56.08,8.53 56.69,7.92 58.32,7.92 58.32,13.82 R25.2
N$45
  Top 0.254: IC5.12 55.88,32.92 56.9,31.9 56.9,9.14 57.1,8.94 T2.1
  Bottom 0.254: T2.1 57.3,8.74 57.3,5.28 70.92,5.28 72.34,3.86 R24.1
N$47  (via drill 0.3)
  Top 0.254: v61.37,19.3 62.79,20.73 62.79,21.54 CHANGE.3
  Bottom 0.254: v61.37,19.3 41.25,19.3 40.03,18.09 38.2,18.09 37.39,17.27 28.65,17.27 28.04,16.66 R23.1
N$48
  Bottom 0.254: R35.1 28.04,19.1 29.46,20.52 56.29,20.52 56.69,20.93 59.74,20.93 61.57,22.76 61.57,26.62 62.79,26.62 CHANGE.1
NOISE
  Top 0.254: R33.2 39.22,45.72 37.8,44.3 37.8,33.93 36.98,33.12 IC4.12
  Bottom 0.254: C11.1 12.6,16.66 10.36,18.9 5.08,18.9 4.88,19.1 4.88,25.81 10.16,25.81 11.18,26.82 25.81,26.82 26.62,27.64 26.62,32.92 IC4.8 26.82,33.12 28.45,34.75 35.15,34.75 36.78,33.12 IC4.12
START_OF_LOOP  (via drill 0.3)
  Top 0.254: IC5.10 50.8,33.12 58.32,40.64 IC5.2 | v79.25,31.5 79.25,20.32 80.47,19.1 R17.1
  Bottom 0.254: v79.25,31.5 79.05,31.29 74.57,31.29 73.36,32.51 73.36,34.75 64.41,34.75 61.98,32.31 61.98,31.29 52.43,31.29 50.8,32.92 IC5.10

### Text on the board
Bottom: Allen Strange | Hal Chamberlin | Inspired | Dieter | by: | Doepfer | Ken Stone | Lunetta | Stanley | Fredkin&Minsky | Muffs | Glass | Navs | &Reich | Nicholas Collins | John | Don Buchla | K.F.W | Cage | Grant Richter
bPlace: Designed in Herne Hill, London, May 2012 by Tom Whitwell | Documentation: musicthing.co.uk/modular/ | Random Sequencer | Rev 2.1 (cap fix) | Sept 2012

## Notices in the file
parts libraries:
SparkFun-Passives: Licensing: CC v3.0 Share-Alike You are welcome to use this library for commercial purposes.
